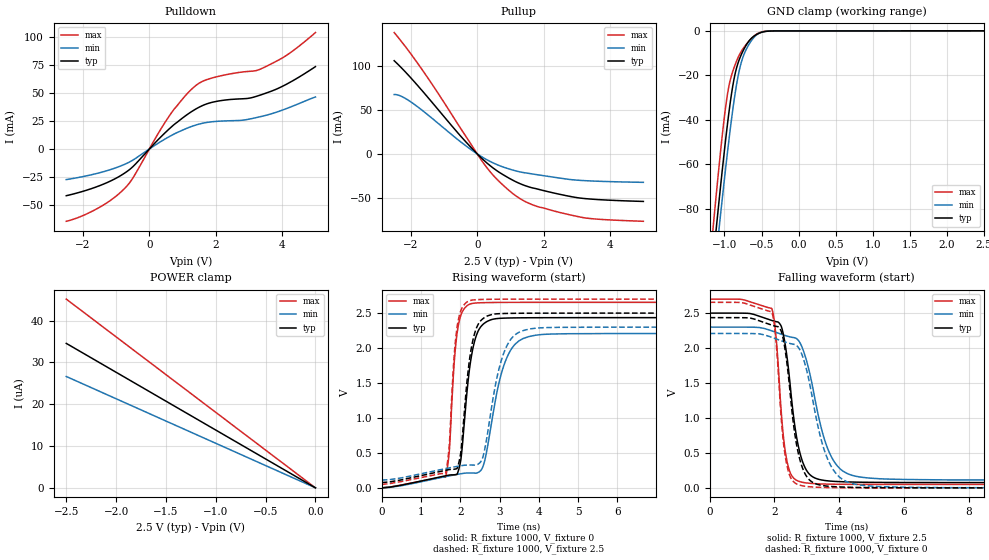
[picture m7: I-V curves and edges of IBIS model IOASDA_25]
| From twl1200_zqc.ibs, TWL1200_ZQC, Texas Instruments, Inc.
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[Model]   IOASDA_25
Model_type  I/O
Vinl=0.875
Vinh=1.625
Enable   Active-Low
Vref =   2.5
Rref =   1M
Cref =   15p
Vmeas =   1.25
| variable   typ   min   max
C_comp   3.70pF   3.05pF   4.62pF
| C_pullup   4.38pF   3.36pF   5.15pF
| C_pulldown   4.38pF   3.64pF   4.88pF
| C_tri-state   3.70pF   3.05pF   4.62pF
[Temperature Range]   40   100   -40
| Ambient temperature   25   85   -40
[Voltage range]   2.5   2.3   2.7
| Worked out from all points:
|   slope of the pulldown table from 0 to 0.375 V, typ, clamps not added: 32.3 ohm
|   slope of the pullup table from 0 to 0.375 V, typ, clamps not added: 29 ohm
|   GND clamp passes 1 mA (typ) near -0.53 V on its own axis
|   rising waveform, R_fixture 1000, V_fixture 0: 20-80 % time 273ps typ, 477ps min, 178ps max; typ from 0.003 V to 2.44 V
|   falling waveform, R_fixture 1000, V_fixture 2.5: 20-80 % time 412ps typ, 692ps min, 270ps max; typ from 2.5 V to 0.078 V
|   rising waveform, R_fixture 1000, V_fixture 2.5: 20-80 % time 262ps typ, 445ps min, 175ps max; typ from 0.078 V to 2.5 V
|   falling waveform, R_fixture 1000, V_fixture 0: 20-80 % time 404ps typ, 670ps min, 266ps max; typ from 2.44 V to 0.003 V
[GND Clamp]
| IOASDA_25
|   Voltage   I(typ)   I(min)   I(max)
-2.5V     -598.9mA   -590.6mA   -610.7mA
-1.15V    -101.8mA   -113.6mA   -87.22mA
-1.105V   -86.79mA   -99.05mA   -71.51mA
-1.065V   -73.75mA   -86.36mA   -58.1mA
-1.005V   -55.04mA   -67.91mA   -39.7mA
-960mV    -42.05mA   -54.72mA   -28.6mA
-900mV    -27.23mA   -38.47mA   -19.48mA
-855mV    -19.12mA   -27.86mA   -15.13mA
-795mV    -12.45mA   -17.04mA   -10.54mA
-735mV    -8.086mA   -10.47mA   -7.334mA
-545mV    -1.273mA   -1.319mA   -1.079mA
2.5V      444.4pA    2.135uA    -3.613uA
[POWER Clamp]
| IOASDA_25
|   Voltage   I(typ)   I(min)   I(max)
-2.5V     34.57uA    26.65uA    45.15uA
-90mV     1.246uA    964.2nA    1.63uA
-60mV     832.2nA    645.4nA    1.086uA
0V        0A         0A         0A
[Pulldown]
| IOASDA_25
|   Voltage   I(typ)   I(min)   I(max)
-2.5V     -41.71mA   -27.32mA   -64.51mA
-1.5V     -32.79mA   -21.26mA   -52.05mA
-720mV    -21.07mA   -13.4mA    -34.48mA
-475mV    -15.21mA   -9.574mA   -24.93mA
640mV     18.99mA    11.63mA    31.11mA
1.085V    29.48mA    17.87mA    47.48mA
1.42V     35.95mA    21.49mA    57.02mA
2.005V    42.31mA    24.55mA    64.16mA
2.8V      44.71mA    25.59mA    68.59mA
3.365V    48.27mA    28.93mA    71.45mA
4.13V     57.72mA    36.01mA    83.47mA
5V        73.38mA    46.31mA    103.7mA
[Pullup]
| IOASDA_25
|   Voltage   I(typ)   I(min)   I(max)
-2.5V     105.6mA    67.26mA    137.5mA
-2.27V    97.06mA    64.99mA    126.8mA
-1.92V    82.86mA    56.85mA    109.3mA
-1.245V   53.26mA    36.76mA    72.47mA
-510mV    20.59mA    13.99mA    29.44mA
30mV      -1.142mA   -741.1uA   -1.752mA
515mV     -17.01mA   -10.84mA   -25.68mA
1.105V    -30.47mA   -18.67mA   -45.9mA
1.42V     -35.67mA   -21.31mA   -53.52mA
1.785V    -39.53mA   -23.44mA   -59.3mA
3.055V    -49.81mA   -29.86mA   -71.19mA
5V        -53.84mA   -32.21mA   -76.35mA
[Ramp]
| IOASDA_25
| variable   typ   min   max
dV/dt_r   1.46/2.78E-10   1.32/4.78E-10   1.59/1.81E-10
dV/dt_f   1.45/4.18E-10   1.31/6.95E-10   1.59/2.72E-10
R_load = 1000
[Rising Waveform]
| IOASDA_25
R_fixture =   1000
C_fixture =   0
L_fixture =   0
V_fixture =   0
V_fixture_min = 0
V_fixture_max = 0
|   Time   V(typ)   V(min)   V(max)
0s        2.798mV    2.924mV    2.735mV
1.625ns   174.8mV    163.1mV    159.1mV
1.72ns    186mV      173.6mV    518.8mV
1.915ns   194.7mV    194.2mV    2.197V
2.315ns   1.979V     215mV      2.639V
2.69ns    2.383V     577.2mV    2.651V
3ns       2.425V     1.538V     2.653V
3.31ns    2.431V     1.995V     2.654V
4.705ns   2.435V     2.205V     2.654V
240ns     2.435V     2.209V     2.654V
[Falling Waveform]
| IOASDA_25
R_fixture =   1000
C_fixture =   0
L_fixture =   0
V_fixture =   2.5
V_fixture_min = 2.3
V_fixture_max = 2.7
|   Time   V(typ)   V(min)   V(max)
0s        2.5V       2.3V       2.7V
1.915ns   2.396V     2.247V     2.568V
2.035ns   2.38V      2.227V     2.228V
2.175ns   2.341V     2.204V     1.312V
2.41ns    1.791V     2.169V     334.8mV
2.815ns   453.3mV    2.052V     87.45mV
3.58ns    106.4mV    643.4mV    56.92mV
4.39ns    86mV       182.8mV    53.02mV
7.32ns    78.46mV    116.5mV    51.9mV
240ns     78.1mV     113.6mV    51.89mV
[Rising Waveform]
| IOASDA_25
R_fixture =   1000
C_fixture =   0
L_fixture =   0
V_fixture =   2.5
V_fixture_min = 2.3
V_fixture_max = 2.7
|   Time   V(typ)   V(min)   V(max)
0s        78.1mV     113.6mV    51.88mV
1.625ns   253mV      277.7mV    212.2mV
1.72ns    264.1mV    288.4mV    608.5mV
1.915ns   276.8mV    309mV      2.283V
2.285ns   2.011V     328.8mV    2.684V
2.645ns   2.446V     621mV      2.696V
2.95ns    2.49V      1.62V      2.699V
3.245ns   2.496V     2.092V     2.699V
4.5ns     2.5V       2.296V     2.7V
240ns     2.5V       2.3V       2.7V
[Falling Waveform]
| IOASDA_25
R_fixture =   1000
C_fixture =   0
L_fixture =   0
V_fixture =   0
V_fixture_min = 0
V_fixture_max = 0
|   Time   V(typ)   V(min)   V(max)
0s        2.435V     2.209V     2.654V
1.915ns   2.329V     2.154V     2.519V
2.035ns   2.313V     2.134V     2.168V
2.165ns   2.278V     2.112V     1.298V
2.4ns     1.727V     2.076V     292.4mV
2.8ns     380.7mV    1.96V      38.91mV
3.565ns   30.96mV    506.1mV    7.75mV
4.37ns    10.56mV    68.91mV    3.875mV
7.285ns   3.16mV     5.707mV    2.754mV
240ns     2.798mV    2.924mV    2.735mV
